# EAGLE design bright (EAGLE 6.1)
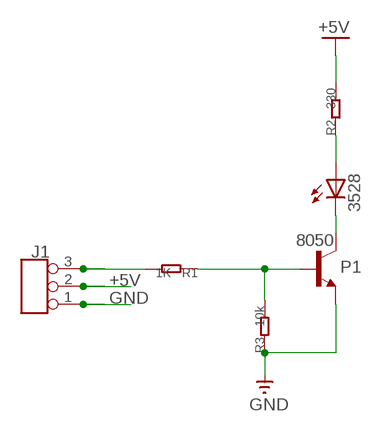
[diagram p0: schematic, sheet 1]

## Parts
3528  LED3528  [3528]
J1  TINKER_3P_DIP  [3P_2.0_DIP]
P1  8050  [SOT23]
R1  1K  R-0603  [R0603]
R2  330  R-0603  [R0603]
R3  10k  R-0603  [R0603]

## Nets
+5V: J1.2 R2.2
GND: J1.1 P1.2(E) R3.1
N$1: J1.3 R1.2
N$2: 3528.1(A) R2.1
N$3: 3528.2(C) P1.3(C)
N$4: P1.1(B) R1.1 R3.2

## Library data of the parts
3528 = example:LED3528
J1 = Connector:TINKER_3P_DIP
P1 = example:8050
R1-R3 = Discrete:R*

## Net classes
0 default: width 0.152 mm, drill 0.305 mm, clearance 0.152 mm

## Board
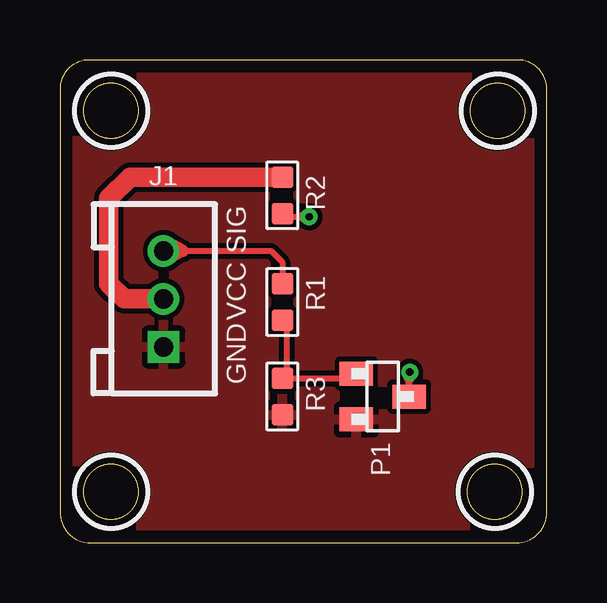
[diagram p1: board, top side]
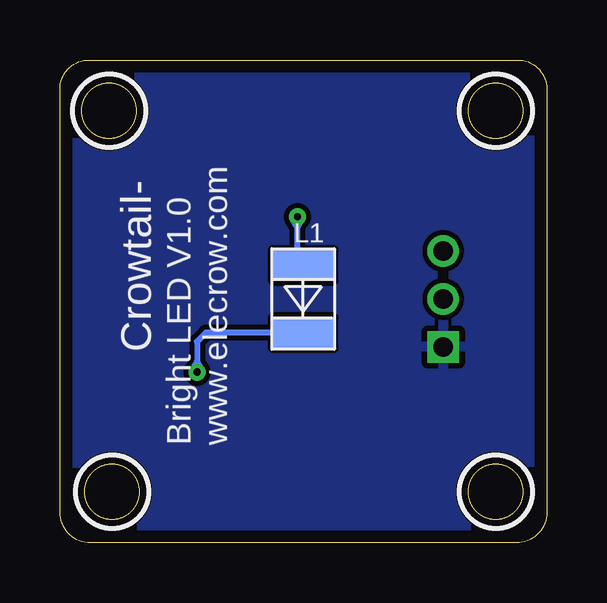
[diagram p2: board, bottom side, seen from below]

Size 20.3 x 20.12 mm. Coordinates in mm from the lower left corner, seen from the top.
Outline: 0,18.91 0,1.27 arc90 1.27,0 19.03,0 arc90 20.3,1.27 20.3,18.91 arc90 19.09,20.12 1.21,20.12 arc90 0,18.91
Outline: circle at 18.26,18 radius 1.14
Outline: circle at 2.13,2.12 radius 1.14
Outline: circle at 18.13,2.12 radius 1.14
Outline: circle at 2.13,18 radius 1.14
Copper layers (1*16): Top 0.035mm / dielectric 1.5mm / Bottom 0.035mm
Design rules "default *": minimum track width 10mil, minimum drill 12mil, track to track 8mil, track to pad 8mil, pad to pad 8mil, via to via 8mil, smd to smd 0mil, copper to edge 20mil, drill to drill 8mil, minimum pad ring 10mil, minimum via ring 8mil, stop-mask expansion 4mil, vias tented up to drill 100mil, thermal gap 10mil
tRestrict: area 16.7,16.5 to 19.8,19.5; area 0.6,0.6 to 3.7,3.6; area 16.6,0.6 to 19.7,3.6; area 0.6,16.5 to 3.7,19.5; area 11.7,5.6 to 13.7,6.5
bRestrict: area 16.7,16.5 to 19.8,19.5; area 0.6,0.6 to 3.7,3.6; area 16.6,0.6 to 19.7,3.6; area 0.6,16.5 to 3.7,19.5

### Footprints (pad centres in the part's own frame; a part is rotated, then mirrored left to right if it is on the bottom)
3528 = smd 1.27 x 2.54: 1 -1.4,0; 2 1.4,0
3P_2.0_DIP = drill 0.8 pad 1.27 square: 1 -2,0 | drill 0.8 pad 1.27: 2 0,0; 3 2,0
SOT23 = smd 1 x 1.4: 1 -0.95,-1.1; 2 0.95,-1.1; 3 0,1.1
R0603 = smd 0.889 x 0.889: 1 -0.762,0; 2 0.762,0

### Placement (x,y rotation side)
3528  10.16,10.16 270 bottom
J1  4.32,10.16 90 top
P1  13.46,6.1 270 top
R1  9.27,10.03 90 top
R2  9.27,14.48 90 top
R3  9.27,6.1 90 top

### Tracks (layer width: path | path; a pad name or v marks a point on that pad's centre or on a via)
+5V
  Top 0.813: J1.2 2.67,10.16 2.03,10.79 2.03,14.35 2.92,15.24 R2.2
GND
  Top 0.406: 12.17,5.33 P1.2
  pour Top: 20.81,20.19 -0.66,20.19 -0.66,-0.38 20.81,-0.38
  pour Bottom: 20.81,20.19 -0.66,20.19 -0.66,-0.25 20.81,-0.25
N$1
  Top 0.254: J1.3 5.12,12.16 8.79,12.16 9.27,11.68 R1.2
  Top 0.406: 9.27,10.67 R1.2
  Top 0.508: 5.12,12.16 | 5.12,12.16 4.52,12.51 | J1.3 4.52,12.51 | 5.12,12.16 | 5.12,12.16 4.52,11.81 | J1.3 4.52,11.81 | 5.12,12.16 4.52,12.51 | 4.52,12.51 | J1.3 4.52,12.51 | 5.12,12.16 4.52,11.81 | J1.3 4.52,11.81 | 5.12,12.16 4.52,12.51 | J1.3 4.52,12.51 | 5.12,12.16 4.52,11.81 | J1.3 4.52,11.81
N$2  (via drill 0.3 pad 0.61)
  Top 0.254: R2.1 9.4,13.59 9.94,13.59 | 9.94,13.59 v10.39,13.59 | 9.94,13.59 | 9.94,13.59 10.28,13.39 | 9.94,13.59 10.28,13.79 | 10.28,13.79 | v10.39,13.59 10.28,13.79 | 9.94,13.59 | 9.94,13.59 | 9.94,13.59 10.28,13.39 | 10.28,13.39 | v10.39,13.59 10.28,13.39 | 9.94,13.59 10.28,13.79 | 9.94,13.59 10.28,13.39 | v10.39,13.59 10.28,13.39 | 9.94,13.59 10.28,13.79 | 10.28,13.79 | v10.39,13.59 10.28,13.79 | 9.94,13.59 10.28,13.39 | v10.39,13.59 10.28,13.39 | 9.94,13.59 10.28,13.79 | v10.39,13.59 10.28,13.79
  Bottom 0.254: 3528.1 10.39,11.79 10.39,13.13 | 10.39,13.13 v10.39,13.59 | 10.39,13.13 | 10.39,13.13 10.59,13.48 | 10.59,13.48 | v10.39,13.59 10.59,13.48 | 10.39,13.13 10.2,13.48 | 10.39,13.13 10.59,13.48 | 10.59,13.48 | 10.39,13.13 10.2,13.48 | 10.2,13.48 | 10.39,13.13 10.59,13.48 | v10.39,13.59 10.59,13.48 | 10.39,13.13 10.2,13.48 | 10.2,13.48 | v10.39,13.59 10.2,13.48 | 10.39,13.13 10.59,13.48 | 10.39,13.13 | 10.39,13.13 10.2,13.48 | v10.39,13.59 10.2,13.48 | 10.39,13.13 10.59,13.48 | v10.39,13.59 10.59,13.48 | 10.39,13.13 10.2,13.48 | v10.39,13.59 10.2,13.48
N$3  (via drill 0.3 pad 0.61)
  Top 0.254: P1.3 14.56,6.66 | 14.56,6.66 14.56,7.09 v14.58,7.11 | 14.56,6.66 14.78,6.99 v14.58,7.11 | 14.56,6.66 14.38,7.01 v14.58,7.11
  Bottom 0.254: 3528.2 14.21,8.76 14.58,8.38 14.58,7.57 | 14.58,7.57 v14.58,7.11 | 14.58,7.57 | 14.58,7.57 14.39,7.23 | 14.58,7.57 14.78,7.23 | 14.78,7.23 | v14.58,7.11 14.78,7.23 | 14.58,7.57 | 14.58,7.57 | 14.58,7.57 14.39,7.23 | 14.39,7.23 | 14.58,7.57 14.39,7.23 | 14.39,7.23 | v14.58,7.11 14.39,7.23 | 14.58,7.57 14.78,7.23 | 14.58,7.57 14.39,7.23 | v14.58,7.11 14.39,7.23 | 14.58,7.57 14.78,7.23 | 14.78,7.23 | v14.58,7.11 14.78,7.23 | 14.58,7.57 14.39,7.23 | v14.58,7.11 14.39,7.23 | 14.58,7.57 14.78,7.23 | v14.58,7.11 14.78,7.23
N$4
  Top 0.254: R3.2 12.17,6.86 P1.1 | 9.46,7.05 9.46,9.08 R1.1
  Top 0.406: 9.46,7.05 R3.2

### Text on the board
tPlace: SIG | VCC | GND
bPlace: Crowtail- | L1 | www.elecrow.com | Bright LED V1.0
